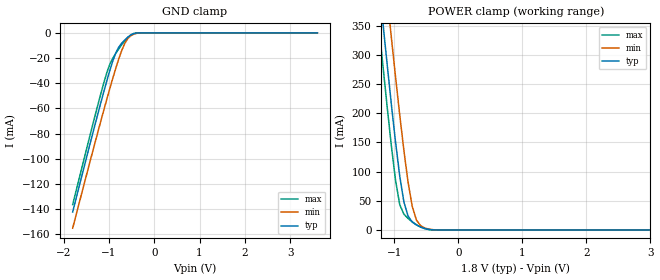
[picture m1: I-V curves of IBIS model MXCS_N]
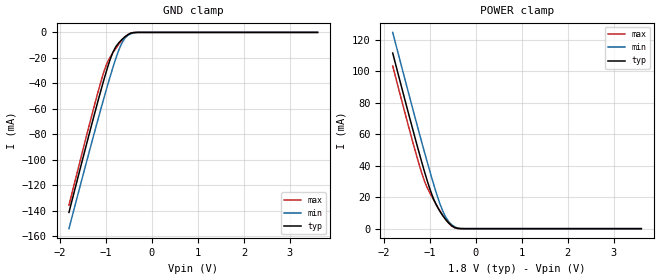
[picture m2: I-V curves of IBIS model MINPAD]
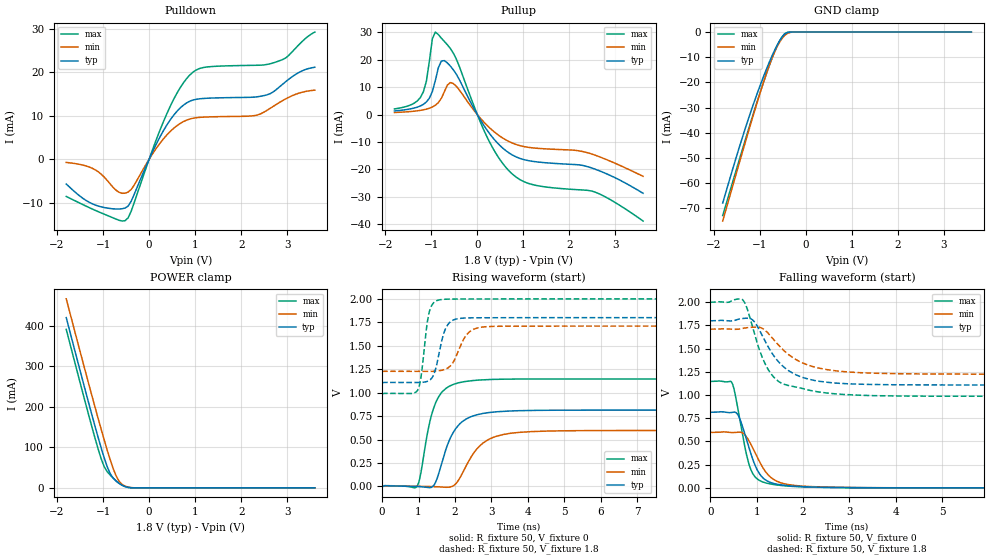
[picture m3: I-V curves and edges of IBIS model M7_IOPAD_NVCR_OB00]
| Created by SiliconSmart  O-2018.09-SP2-3
[IBIS Ver]   4.0
[File Name]   as1a04wa_rev1p4.ibs
[File Rev]   1.4
[Date]   Thursday Mar 21 2024
|[Source]   Avalanche Team
|[Notes]   Generated IBIS models from Silicon Smart
|[Rev 1.0]  Initial Release based on extracted netlist
|   Characterization
|[Rev 1.1]  Update Package RLC
|[Rev 1.2]  Recharacterize MIOPAD with Hspice run in high accuracy mode
|[Rev 1.3]  Recharacterize with parameters aligned in datasheet
|[Rev 1.4]  Update the pin to the package pinout assignment
|[Disclaimer]   THE MODEL LIBRARIES ARE PROVIDED AS IS.
|[Copyright]   Copyright 2019, Avalanche Technology., All Rights Reserved
[Component]   AS10xxA04_WSON
[Manufacturer] Avalanche Technology
| CONTENT :
| This file contains IBIS MODEL for PSRAM device
| AS1016A04
| USAGE :
| The models are derived for the 1.71V to 2.0V I/O Operation.
| Temperatures for model generation: typ: 25, max: -40, min: 125
| Voltages : typ: 1.8V, min: 1.71V, max: 2.0V
| PACKAGES SUPPORTED :
| 8-pad WSON (5.0mm x 6.0mm)
| VERIFICATION :
| Errors  : 0
| Warnings: 31
| All warnings due to non-monotonic data
[Package]
|variable   typ   min   max
R_pkg   8.90E-04   8.89E-04  8.91E-04
L_pkg   1.185E-09  1.18E-09  1.19E-09
C_pkg   2.30E-13   2.21E-13  2.39E-13
[Pin]   signal_name   model_name   R_pin   L_pin   C_pin
1   CS#   MXCS_N   1.05E-01  1.35E-09  9.16E-14
2   SO   MIOPAD   1.05E-01  1.35E-09  9.16E-14
3   WP#   MIOPAD   1.05E-01  1.35E-09  9.16E-14
5   SI   MIOPAD   3.75E-02  3.89E-10  4.24E-14
6   CLK   MINPAD   3.75E-02  3.89E-10  4.24E-14
7   IO_3   MIOPAD   3.75E-02  3.89E-10  4.24E-14
4   VSS   GND   NA   NA   NA
8   VCC   POWER   NA   NA   NA
[Model Selector] MIOPAD
| Model Description
M0_IOPAD_NVCR_OB07   20 Ohms drv strength
M1_IOPAD_NVCR_OB06   30 Ohms drv strength
M2_IOPAD_NVCR_OB05   60 Ohms drv strength
M3_IOPAD_NVCR_OB04   45 Ohms drv strength
M4_IOPAD_NVCR_OB03   70 Ohms drv strength
M5_IOPAD_NVCR_OB02   90 Ohms drv strength
M6_IOPAD_NVCR_OB01   120 Ohms drv strength
M7_IOPAD_NVCR_OB00   45 Ohms drv strength
| Models and submodels in the file (10): MXCS_N (Input), MINPAD (Input), M7_IOPAD_NVCR_OB00 (I/O), M3_IOPAD_NVCR_OB04 (I/O), M5_IOPAD_NVCR_OB02 (I/O), M1_IOPAD_NVCR_OB06 (I/O), M6_IOPAD_NVCR_OB01 (I/O), M2_IOPAD_NVCR_OB05 (I/O), M4_IOPAD_NVCR_OB03 (I/O), M0_IOPAD_NVCR_OB07 (I/O)
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| XCS_N
[Model] MXCS_N
Model_type Input
Enable   Active-High
Vinl  =  0.54
Vinh  =  1.26
| Capacitance  typ   min   max
C_comp   3.084351e-12   2.813138e-12   3.417919e-12
| Variables   typ   min   max
[GND Clamp Reference]   0   0   0
[POWER Clamp Reference]   1.8   1.71   2
[Pulldown Reference]   0   0   0
[Pullup Reference]   1.8   1.71   2
[Temperature Range]   25   125   -40
[Voltage Range]   1.8   1.71   2
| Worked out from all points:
|   GND clamp passes 1 mA (typ) near -0.48 V on its own axis
|   POWER clamp passes 1 mA (typ) near -0.46 V on its own axis
[GND Clamp]
| Voltage   I(typ)   I(min)   I(max)
-1.8V     -142.2mA   -155mA     -136.3mA
-1.303V   -72.38mA   -86.68mA   -65.31mA
-1.043V   -37.59mA   -52.15mA   -31.14mA
-977.6mV  -29.52mA   -43.82mA   -24.56mA
-912.4mV  -22.07mA   -35.71mA   -19.91mA
-847.2mV  -15.78mA   -27.9mA    -16.17mA
-782.1mV  -11.28mA   -20.54mA   -12.65mA
-651.7mV  -5.669mA   -8.443mA   -6.326mA
-521.4mV  -1.817mA   -2.372mA   -1.753mA
-391mV    -121.1uA   -342.2uA   -61.96uA
-260.7mV  -1.429uA   -15.13uA   -173.3nA
3.6V      0A         0A         0A
[POWER Clamp]
| Voltage   I(typ)   I(min)   I(max)
-1.8V     1.062A     1.175A     991.6mA
-1.238V   424.5mA    540.7mA    351.4mA
-1.173V   353.2mA    469.3mA    280.1mA
-1.043V   215.2mA    329.7mA    144.3mA
-977.6mV  150.6mA    262.1mA    85.02mA
-912.4mV  92.52mA    197.1mA    43.53mA
-847.2mV  47.97mA    136mA      27.04mA
-782.1mV  23.77mA    81.82mA    19.63mA
-716.9mV  13.61mA    40.38mA    13.92mA
-651.7mV  8.604mA    16.99mA    8.943mA
-325.9mV  22.75uA    117uA      9.962uA
3.6V      0A         0A         0A
| INPAD
[Model] MINPAD
Model_type Input
Enable   Active-High
Vinl  =  0.54
Vinh  =  1.26
| Capacitance  typ   min   max
C_comp   2.700843e-12   2.498345e-12   2.944515e-12
| Variables   typ   min   max
[GND Clamp Reference]   0   0   0
[POWER Clamp Reference]   1.8   1.71   2
[Pulldown Reference]   0   0   0
[Pullup Reference]   1.8   1.71   2
[Temperature Range]   25   125   -40
[Voltage Range]   1.8   1.71   2
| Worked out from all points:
|   GND clamp passes 1 mA (typ) near -0.48 V on its own axis
|   POWER clamp passes 1 mA (typ) near -0.47 V on its own axis
[GND Clamp]
| Voltage   I(typ)   I(min)   I(max)
-1.8V     -141.2mA   -153.9mA   -135.5mA
-1.303V   -71.9mA    -86.07mA   -64.94mA
-1.043V   -37.35mA   -51.79mA   -30.99mA
-977.6mV  -29.34mA   -43.53mA   -24.44mA
-912.4mV  -21.94mA   -35.48mA   -19.81mA
-847.2mV  -15.7mA    -27.72mA   -16.09mA
-782.1mV  -11.23mA   -20.42mA   -12.58mA
-651.7mV  -5.65mA    -8.408mA   -6.299mA
-521.4mV  -1.813mA   -2.367mA   -1.748mA
-391mV    -121uA     -342uA     -61.94uA
-260.7mV  -1.429uA   -15.13uA   -173.3nA
3.6V      0A         0A         0A
[POWER Clamp]
| Voltage   I(typ)   I(min)   I(max)
-1.8V     111.7mA    124.8mA    103.4mA
-1.369V   63.57mA    76.61mA    55.54mA
-1.238V   49.53mA    62.37mA    41.97mA
-1.108V   36.07mA    48.41mA    30.06mA
-977.6mV  23.92mA    34.89mA    21.88mA
-912.4mV  18.87mA    28.39mA    18.39mA
-782.1mV  11.36mA    16.45mA    11.73mA
-651.7mV  5.917mA    7.437mA    5.926mA
-521.4mV  1.955mA    2.53mA     1.736mA
-391mV    174.8uA    429uA      115.2uA
-260.7mV  2.189uA    21.34uA    482.3nA
3.6V      0A         0A         0A
[Model] M7_IOPAD_NVCR_OB00
Model_type I/O
Enable   Active-High
Vinl  =  0.54
Vinh  =  1.26
Vmeas =  0.9
Cref  =  30e-12
| Capacitance  typ   min   max
C_comp   3.869840e-12   3.575244e-12   4.229518e-12
| Variables   typ   min   max
[GND Clamp Reference]   0   0   0
[POWER Clamp Reference]   1.8   1.71   2
[Pulldown Reference]   0   0   0
[Pullup Reference]   1.8   1.71   2
[Temperature Range]   25   125   -40
[Voltage Range]   1.8   1.71   2
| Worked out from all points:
|   slope of the pulldown table from 0 to 0.27 V, typ, clamps not added: 46.6 ohm
|   slope of the pullup table from 0 to 0.27 V, typ, clamps not added: 38.6 ohm
|   GND clamp passes 1 mA (typ) near -0.46 V on its own axis
|   POWER clamp passes 1 mA (typ) near -0.44 V on its own axis
|   falling waveform, R_fixture 50, V_fixture 0: 20-80 % time 347ps typ, 425ps min, 280ps max; typ from 0.814 V to 0 V
|   falling waveform, R_fixture 50, V_fixture 1.8: 20-80 % time 649ps typ, 775ps min, 500ps max; typ from 1.8 V to 1.1 V
|   rising waveform, R_fixture 50, V_fixture 0: 20-80 % time 520ps typ, 650ps min, 397ps max; typ from 0 V to 0.814 V
|   rising waveform, R_fixture 50, V_fixture 1.8: 20-80 % time 256ps typ, 366ps min, 184ps max; typ from 1.1 V to 1.8 V
[GND Clamp]
| Voltage   I(typ)   I(min)   I(max)
-1.8V     -67.84mA   -74.98mA   -72.81mA
-1.499V   -49.26mA   -55.7mA    -54.28mA
-1.303V   -37.87mA   -43.36mA   -42.4mA
-1.043V   -23.96mA   -27.4mA    -27.1mA
-847.2mV  -14.58mA   -16.27mA   -16.36mA
-716.9mV  -8.973mA   -9.798mA   -9.837mA
-651.7mV  -6.447mA   -7.048mA   -6.896mA
-521.4mV  -2.255mA   -2.801mA   -2.141mA
-456.2mV  -849.3uA   -1.361mA   -679.4uA
-391mV    -172uA     -473.2uA   -88.88uA
-260.7mV  -2.088uA   -22.04uA   -254.3nA
3.6V      0A         0A         0A
[POWER Clamp]
| Voltage   I(typ)   I(min)   I(max)
-1.8V     419.8mA    466.1mA    390.9mA
-1.303V   205.4mA    252.8mA    175.7mA
-1.043V   98.85mA    144.9mA    72.14mA
-977.6mV  74.56mA    119mA      52.56mA
-912.4mV  52.76mA    93.87mA    40.16mA
-847.2mV  35.48mA    69.92mA    31.71mA
-716.9mV  16.42mA    29.44mA    17.31mA
-651.7mV  10.9mA     16.21mA    11.28mA
-586.6mV  6.514mA    8.5mA      6.386mA
-456.2mV  1.168mA    1.854mA    921.1uA
-325.9mV  31.2uA     159.5uA    13.68uA
3.6V      0A         0A         0A
[Pulldown]
| Voltage   I(typ)   I(min)   I(max)
-1.8V     -5.69mA    -732.8uA   -8.548mA
-1.173V   -10.5mA    -2.407mA   -11.73mA
-716.9mV  -11.43mA   -7.123mA   -13.76mA
-521.4mV  -11.21mA   -7.798mA   -14.11mA
-391mV    -9.672mA   -6.953mA   -11.98mA
372.4mV   7.658mA    5.437mA    10.17mA
869mV     13.26mA    9.198mA    19.2mA
1.179V    13.97mA    9.684mA    21.08mA
2.283V    14.28mA    10.02mA    21.59mA
2.766V    16.04mA    12.62mA    22.39mA
3.248V    19.92mA    15.17mA    26.27mA
3.6V      21.15mA    15.89mA    29.24mA
[Pullup]
| Voltage   I(typ)   I(min)   I(max)
-1.8V     1.352mA    789.5uA    2.099mA
-1.238V   3.177mA    1.572mA    6.26mA
-1.108V   4.622mA    2.015mA    12.15mA
-977.6mV  8.411mA    2.79mA     27.68mA
-912.4mV  12.48mA    3.432mA    30.16mA
-782.1mV  19.57mA    5.979mA    27.92mA
-521.4mV  16.37mA    11.35mA    22.45mA
186.2mV   -5.049mA   -3.49mA    -7.284mA
744.8mV   -14.56mA   -10.25mA   -21.44mA
1.241V    -17.12mA   -12.19mA   -25.69mA
2.559V    -19.89mA   -14.78mA   -28.27mA
3.6V      -28.69mA   -22.5mA    -38.81mA
[Ramp]
dV/dt_r   0.488568/0.519945n  0.3582/0.649804n  0.687926/0.397312n
dV/dt_f   0.417076/0.649039n  0.291154/0.774597n  0.608145/0.500349n
R_load = 50
[Falling Waveform]
R_fixture = 50
V_fixture = 0
V_fixture_min = 0
V_fixture_max = 0
| Time   V(typ)   V(min)   V(max)
0s        814.3mV    597mV      1.147V
474ps     813.8mV    595.5mV    1.125V
599.7ps   783.2mV    599.8mV    837.3mV
776.9ps   525.9mV    551.6mV    365.8mV
857.5ps   394.6mV    485.8mV    218.7mV
948.2ps   264.1mV    396.3mV    129.1mV
1.169ns   92.84mV    190.4mV    56.83mV
1.546ns   30.54mV    50.91mV    24.51mV
3.59ns    987.2uV    1.63mV     780.3uV
21.88ns   242.1nV    1.102uV    249.8nV
[Falling Waveform]
R_fixture = 50
V_fixture = 1.8
V_fixture_min = 1.71
V_fixture_max = 2
| Time   V(typ)   V(min)   V(max)
0s        1.8V       1.71V      2V
684.9ps   1.824V     1.717V     2.031V
791.9ps   1.828V     1.726V     1.935V
954.3ps   1.787V     1.732V     1.656V
1.128ns   1.633V     1.716V     1.397V
1.355ns   1.433V     1.605V     1.2V
1.831ns   1.222V     1.387V     1.089V
2.549ns   1.136V     1.271V     1.02V
4.583ns   1.109V     1.227V     987.9mV
21.88ns   1.105V     1.225V     986.4mV
[Rising Waveform]
R_fixture = 50
V_fixture = 0
V_fixture_min = 0
V_fixture_max = 0
| Time   V(typ)   V(min)   V(max)
0s        74.44nV    863.5nV    131.9nV
944.2ps   468.1uV    1.924mV    -6.144mV
1.049ns   -1.961mV   1.531mV    113mV
1.314ns   -12.28mV   -427.4uV   697.4mV
1.509ns   84.57mV    -3.045mV   925.6mV
1.949ns   574.2mV    5.58mV     1.087V
2.418ns   740.7mV    298.7mV    1.126V
3.009ns   791.1mV    517.2mV    1.141V
4.315ns   811.6mV    588.4mV    1.146V
21.88ns   814.3mV    597mV      1.147V
[Rising Waveform]
R_fixture = 50
V_fixture = 1.8
V_fixture_min = 1.71
V_fixture_max = 2
| Time   V(typ)   V(min)   V(max)
0s        1.105V     1.225V     986.4mV
973.3ps   1.108V     1.227V     1.024V
1.065ns   1.109V     1.226V     1.158V
1.296ns   1.131V     1.227V     1.861V
1.443ns   1.219V     1.229V     1.968V
1.614ns   1.514V     1.237V     1.992V
1.902ns   1.764V     1.297V     1.998V
2.365ns   1.797V     1.637V     1.999V
2.86ns    1.799V     1.703V     1.999V
21.88ns   1.8V       1.71V      2V
